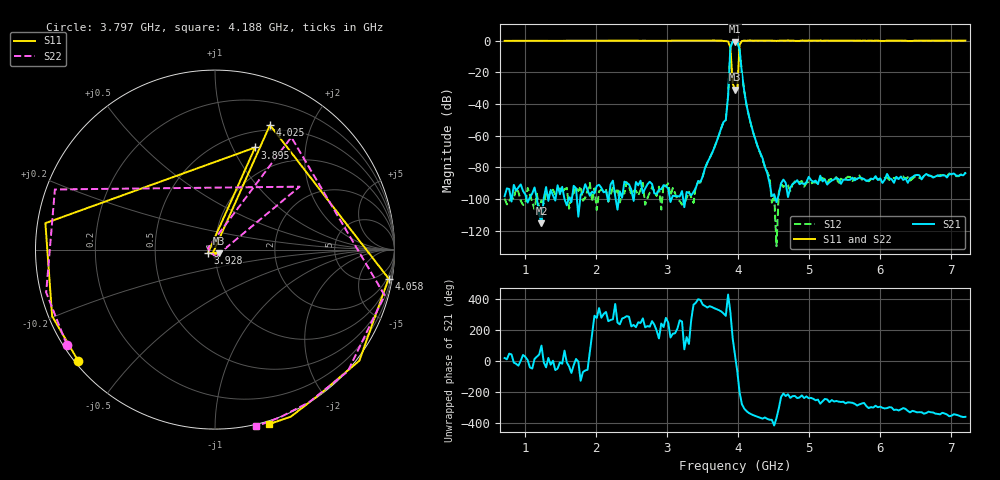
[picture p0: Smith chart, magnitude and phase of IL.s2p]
!Agilent Technologies,E8364B,MY43040703,A.07.50.48
!Agilent E8364B: A.07.50.48
!Date: Wednesday, April 10, 2024 15:18:29
!Correction: S11(Full 2 Port(1,2))
!S21(Full 2 Port(1,2))
!S12(Full 2 Port(1,2))
!S22(Full 2 Port(1,2))
!S2P File: Measurements: S11, S21, S12, S22:
# Hz S  dB  R 50
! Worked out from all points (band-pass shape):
!   201 points, 710 MHz to 7.21 GHz, reference 50 ohm
!   highest |S21| = -0.46 dB at 3.96 GHz (marker M1); lowest = -115.4 dB at 1.23 GHz (marker M2)
!   |S21| within 3 dB of the highest: 3.9 GHz to 4.011 GHz (111.2 MHz wide, 2.81 % of centre)
!   lowest |S11| = -30.9 dB at 3.96 GHz (marker M3), VSWR 1.06, Z = 52 - j2.11 ohm
!   |S11| at or under -10 dB: 3.903 GHz to 4.016 GHz (113.1 MHz wide, 2.86 % of centre)
!   |S22| runs from -27.7 to 0.2 dB; largest |S21 - S12| = 0.011
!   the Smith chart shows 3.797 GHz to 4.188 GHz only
!   S11 on the Smith chart (normalised r, x): 3.797 GHz: 0.01, -0.36; 3.895 GHz: 0.68, +1.23; 3.928 GHz: 0.92, -0.04; 4.025 GHz: 0.44, +1.44; 4.058 GHz: 1, -12; 4.188 GHz: -0.03, -1.35
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7.1e8  -0.05 122.1  -98.20 18.0  -99.71 65.2  -0.09 119.6
1.23e9  -0.02 81.4  -115.37 98.0  -100.79 -4.7  -0.08 78.1
1.815e9  0.06 37.6  -95.73 -72.3  -101.05 -89.0  0.01 33.3
2.3025e9  0.01 2.6  -106.74 -113.9  -93.15 -86.5  0.04 -1.8
2.8875e9  0.04 -38.8  -94.04 143.9  -92.15 -107.8  -0.01 -43.2
3.5375e9  0.11 -91.3  -80.30 -7.2  -80.76 -2.6  0.14 -95.1
3.7e9  0.08 -113.3  -63.76 -27.5  -63.89 -26.5  0.13 -118.5
3.7975e9  -0.15 -140.8  -51.36 -54.8  -51.34 -54.7  -0.16 -147.2
3.83e9  -0.17 -157.8  -50.09 -70.8  -50.08 -70.4  -0.26 -165.8
3.8625e9  -0.39 171.1  -34.94 66.7  -34.89 66.7  -0.42 159.4
3.895e9  -4.28 68.6  -4.02 -46.6  -3.94 -46.6  -4.62 36.6
3.9275e9  -26.99 -153.3  -0.60 142.5  -0.51 142.1  -27.01 -94.2
3.96e9  -30.89 -45.4  -0.46 34.8  -0.39 34.7  -27.16 -83.5
3.9925e9  -30.67 -120.0  -0.51 -68.5  -0.47 -68.4  -27.74 170.4
4.025e9  -2.40 66.2  -5.58 156.5  -5.48 156.2  -2.42 55.8
4.0575e9  -0.17 -9.5  -20.56 80.5  -20.44 80.6  -0.19 -15.1
4.09e9  0.13 -37.6  -31.67 52.5  -31.62 52.4  0.03 -42.5
4.1875e9  0.16 -72.9  -53.09 16.5  -53.20 16.4  0.10 -76.9
4.3825e9  0.09 -100.8  -79.81 -4.6  -79.84 -18.0  0.15 -105.5
5.065e9  0.11 -151.9  -89.12 115.2  -89.56 113.2  0.08 -154.8
6.1375e9  0.08 148.8  -86.74 61.5  -87.95 62.8  0.04 144.0
7.21e9  0.15 92.9  -83.62 -0.4  -83.69 -0.3  0.17 88.4
